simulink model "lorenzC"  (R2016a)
settings: Solver=ode45  StartTime=0.0  StopTime=50  MaxStep=0.01  RelTol=1e-3
InitFcn:
  | init_lorenzC
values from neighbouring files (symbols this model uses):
  a = 10    [init_lorenzC.m]
  b = zeros(N, 1)    [fourierrechteck.m]    (also in init_lorenzC.m = 28; init_pendelStange.m = 0.2)
  c = 8/3    (= 2.66666666667)    [init_lorenzC.m]
  phi = block.InputPort(1).Data    [sfun_pendelstangeanim.m]
undefined symbols (not defined in the file or in its folder): psi, theta, xlims, ylims, zlims
libraries: simulink x3

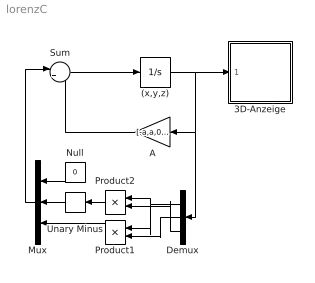
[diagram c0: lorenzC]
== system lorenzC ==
  (x,y,z) : Integrator  InitialCondition=[15 15 15]
  3D-Anzeige : Subsystem
  A : Gain  Gain=[-a,a,0; b,-1,0; 0,0,-c]  Multiplication=Matrix(K*u)
  Demux : Demux  Outputs=3
  Mux : Mux  Inputs=3
  Null : Constant  Value=0
  Product1 : Product
  Product2 : Product
  Sum : Sum  Inputs=|++
  Unary Minus : UnaryMinus
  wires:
  (x,y,z)/1 -> A/1, Demux/1, 3D-Anzeige/1(In)
  A/1 -> Sum/2
  Sum/1 -> (x,y,z)/1
  Product1/1 -> Mux/3
  Null/1 -> Mux/1
  Unary Minus/1 -> Mux/2
  Product2/1 -> Unary Minus/1
  Demux/1 -> Product2/1, Product1/1
  Demux/3 -> Product2/2
  Demux/2 -> Product1/2
  Mux/1 -> Sum/1

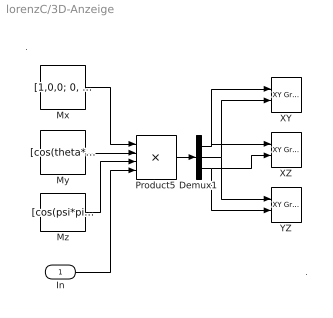
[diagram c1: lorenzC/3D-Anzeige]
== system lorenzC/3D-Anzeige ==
  note: .
  note: .
  In : Inport
  Demux1 : Demux  Outputs=3
  Mx : Constant  Value=[1,0,0; 0, cos(phi*pi/180), -sin(phi*pi/180); 0, sin(phi*pi/180), cos(phi*pi/180)]
  My : Constant  Value=[cos(theta*pi/180),0, sin(theta*pi/180); 0,1,0; -sin(theta*pi/180),0,cos(theta*pi/180)]
  Mz : Constant  Value=[cos(psi*pi/180),-sin(psi*pi/180), 0; sin(psi*pi/180), cos(psi*pi/180), 0; 0,0,1]
  Product5 : Product  Inputs=4  Multiplication=Matrix(*)
  XY : simulink/Sinks/XY Graph  xmin=xlims(1)  xmax=xlims(2)  ymin=ylims(1)  ymax=ylims(2)  st=-1
  XZ : simulink/Sinks/XY Graph  xmin=xlims(1)  xmax=xlims(2)  ymin=zlims(1)  ymax=zlims(2)  st=-1
  YZ : simulink/Sinks/XY Graph  xmin=ylims(1)  xmax=ylims(2)  ymin=zlims(1)  ymax=zlims(2)  st=-1
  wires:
  Demux1/2 -> XY/2, YZ/1
  Demux1/3 -> XZ/2, YZ/2
  Product5/1 -> Demux1/1
  Mz/1 -> Product5/3
  My/1 -> Product5/2
  Mx/1 -> Product5/1
  In/1 -> Product5/4
  Demux1/1 -> XY/1, XZ/1
